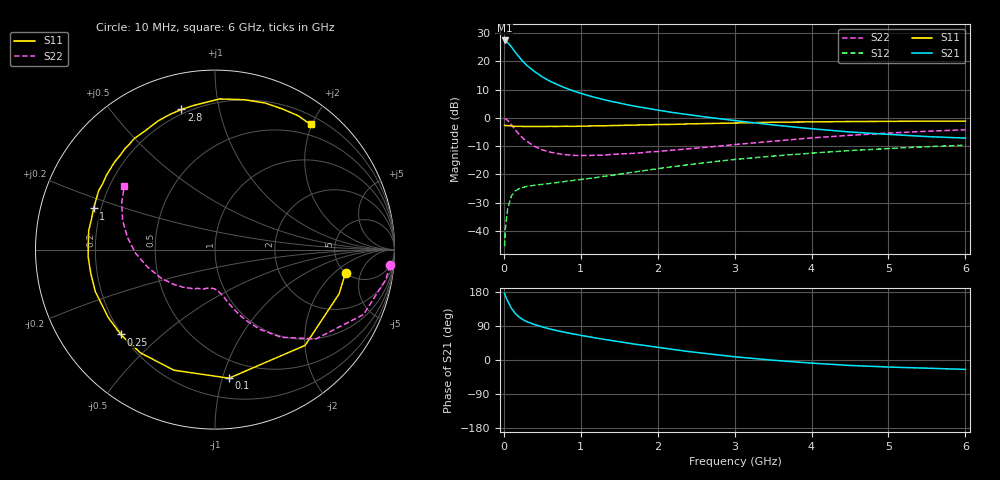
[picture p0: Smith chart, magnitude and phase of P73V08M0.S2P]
! SIEMENS Small Signal Semiconductors
! BFP196
! Si NPN RF Bipolar Junction Transistor in SOT143
! VCE = 3 V  IC = 8 mA
! Common Emitter S-Parameters:  May  1996
# GHz  S  MA  R  50
!  f  S11  S21  S12  S22
! GHz  MAG  ANG  MAG  ANG  MAG  ANG  MAG  ANG
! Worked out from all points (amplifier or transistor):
!   36 points, 10 MHz to 6 GHz, reference 50 ohm
!   highest |S21| = 27.4 dB at 10 MHz (marker M1)
!   |S21| within 3 dB of that: start of sweep to 117.8 MHz
!   unconditionally stable (mu >= 1): 932 MHz to 3.242 GHz
!   at 250 MHz: K = 0.34, MSG = 22.2 dB, |S12| = -24.5 dB
!   at 1.4 GHz: K = 1.16, MAG = 10.7 dB, |S12| = -20.3 dB
!   at 6 GHz: K = 0.98, MSG = 1.3 dB, |S12| = -9.6 dB
!   S11 on the Smith chart (normalised r, x): 10 MHz: 4.98, -2.84; 100 MHz: 0.35, -1.05; 250 MHz: 0.20, -0.37; 1 GHz: 0.17, +0.16; 2.8 GHz: 0.18, +0.77; 6 GHz: 0.33, +1.98
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0.01  0.7386 -10.1  23.43 175.7  0.0054 85.2  0.9788 -5.1
0.02  0.7341 -19.7  22.8 169.3  0.0111 81.1  0.9666 -9.9
0.05  0.7324 -46.8  21.53 155.2  0.0251 67.5  0.9031 -23.6
0.1  0.7207 -83.8  17.92 136.0  0.0422 52.5  0.7509 -41.5
0.15  0.7099 -108.8  14.41 122.4  0.0512 42.7  0.6126 -52.9
0.2  0.7097 -125.9  11.92 113.1  0.0563 36.6  0.5102 -60.6
0.25  0.7068 -138.0  9.888 106.2  0.0593 33.2  0.4346 -66.0
0.3  0.7047 -147.4  8.493 101.1  0.0616 31.2  0.3853 -69.7
0.4  0.7065 -160.7  6.59 93.4  0.0645 29.8  0.3135 -75.3
0.5  0.7048 -169.4  5.309 87.3  0.0669 29.5  0.2719 -79.1
0.6  0.7079 -176.9  4.465 81.8  0.0695 30.1  0.2486 -82.4
0.7  0.707 176.6  3.856 77.0  0.0722 31.3  0.2339 -85.2
0.8  0.7118 171.4  3.385 72.8  0.0754 32.7  0.2242 -88.3
1  0.7143 161.3  2.722 65.1  0.0815 35.4  0.2164 -93.7
1.1  0.7183 157.4  2.482 61.5  0.0849 36.5  0.2173 -96.6
1.6  0.7424 138.9  1.712 45.1  0.1061 40.9  0.2338 -110.9
2.2  0.7682 120.1  1.244 27.9  0.1375 41.4  0.2699 -127.8
2.8  0.8028 103.5  0.97 13.1  0.1725 38.2  0.3177 -146.1
3.5  0.8397 88.3  0.751 -0.6  0.2117 31.5  0.3874 -165.3
4.5  0.8631 71.2  0.564 -14.4  0.2645 20.6  0.4933 171.9
5.5  0.8777 58.3  0.468 -21.6  0.3096 8.9  0.5816 153.3
6  0.8778 52.6  0.44 -24.8  0.3294 2.5  0.6169 145.0
